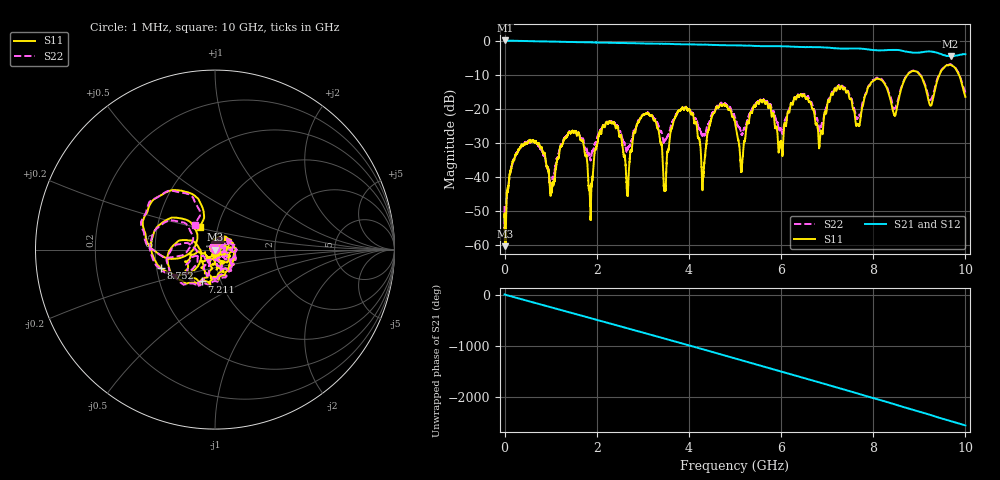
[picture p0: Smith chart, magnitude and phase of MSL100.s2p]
! 3/21/2017 9:29:37 AM
! F:\HUSERTL_20170321\MSL100.S2P
! CHANNEL.1
! TR.MEASUREMENT
! CORRECTED.DATA
# GHZ S RI R 50.0
! FREQ.GHZ  S11RE  S11IM  S31RE  S31IM  S13RE  S13IM  S33RE  S33IM
!; PortSelection: Port_13
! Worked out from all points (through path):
!   10000 points, 1 MHz to 10 GHz, reference 50 ohm
!   highest |S21| = 0.03 dB at 10 MHz (marker M1); lowest = -4.6 dB at 9.678 GHz (marker M2)
!   group delay of S21, straight-line fit = 709 ps
!   lowest |S11| = -60.3 dB at 19 MHz (marker M3), VSWR 1.00, Z = 50 - j0.0924 ohm
!   |S11| at or under -10 dB: start of sweep to 8.746 GHz; 9.011 GHz to 9.438 GHz (427 MHz wide, 4.63 % of centre); 9.861 GHz to end of sweep
!   |S22| runs from -58.9 to -6.9 dB; largest |S21 - S12| = 0.043
!   S11 on the Smith chart (normalised r, x): 1 MHz: 1.01, +0.00; 7.211 GHz: 0.81, -0.30; 8.752 GHz: 0.53, -0.12; 10 GHz: 0.81, +0.20
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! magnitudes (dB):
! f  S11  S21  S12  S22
! 1 MHz  -50.9  0.0  0.0  -53.4
! 10 MHz  -56.6  0.0  0.0  -52.6
! 19 MHz  -60.3  0.0  0.0  -55.2
! 373 MHz  -30.5  -0.1  -0.1  -30.8
! 1.025 GHz  -43.6  -0.3  -0.3  -42.6
! 1.668 GHz  -29.3  -0.5  -0.5  -28.7
! 1.863 GHz  -50.5  -0.5  -0.5  -35.0
! 2.175 GHz  -25.4  -0.6  -0.6  -24.8
! 2.665 GHz  -44.9  -0.7  -0.8  -31.9
! 2.943 GHz  -22.8  -0.8  -0.8  -22.9
! 3.334 GHz  -25.9  -0.9  -0.9  -24.8
! 3.477 GHz  -42.7  -0.9  -0.9  -29.4
! 3.816 GHz  -20.4  -1.1  -1.1  -20.3
! 4.308 GHz  -40.1  -1.2  -1.2  -27.4
! 4.571 GHz  -20.6  -1.3  -1.3  -20.3
! 5.001 GHz  -24.1  -1.4  -1.4  -22.4
! 6.667 GHz  -19.6  -1.9  -2.0  -18.3
! 7.211 GHz  -14.3  -2.3  -2.3  -14.2
! 8.334 GHz  -15.5  -2.8  -2.8  -15.0
! 8.752 GHz  -9.9  -3.3  -3.3  -9.8
! 9.678 GHz  -7.1  -4.6  -4.6  -6.9
! 10 GHz  -16.5  -4.0  -4.0  -15.3
